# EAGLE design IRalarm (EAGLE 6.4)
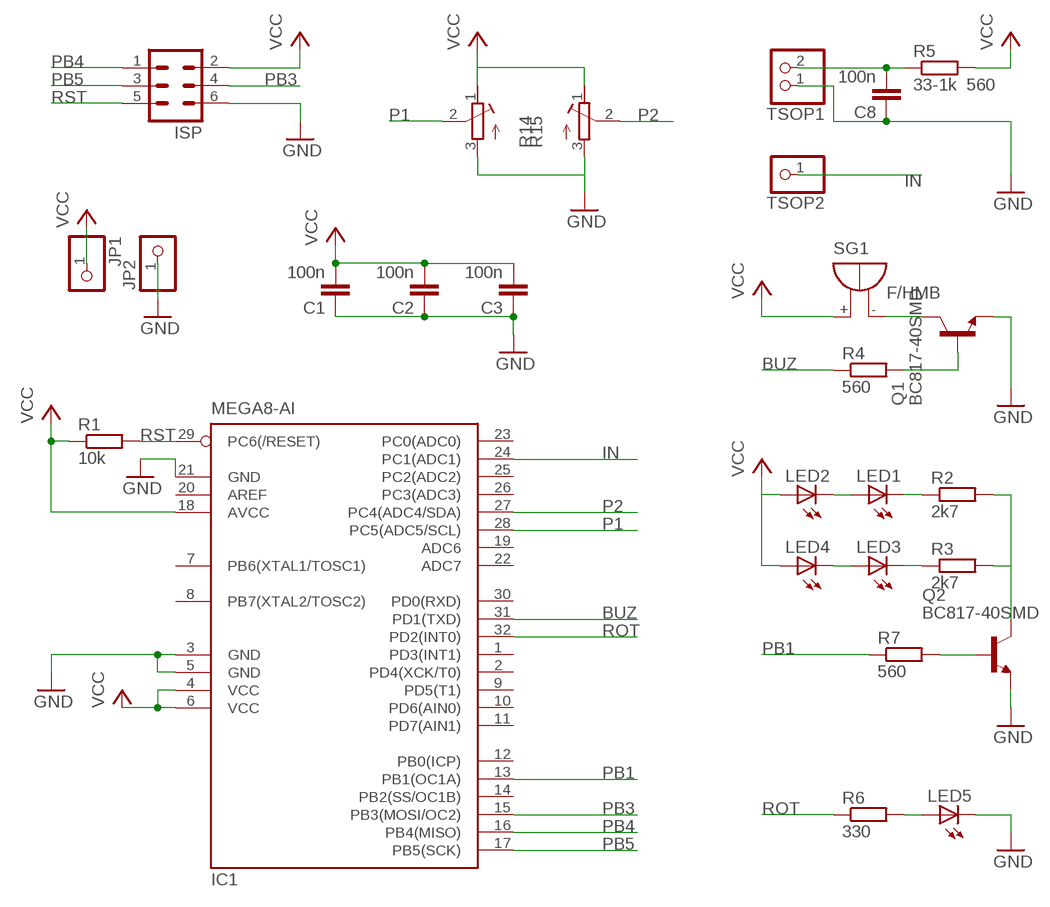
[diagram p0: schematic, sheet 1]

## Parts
C1  100n  C-EUC0805  [C0805]
C2  100n  C-EUC0805  [C0805]
C3  100n  C-EUC0805  [C0805]
C8  100n  C-EUC0805  [C0805]
IC1  MEGA8-AI  [TQFP32-08]
ISP  ML6  [ML6]
JP1  PINHD-1X1  [1X01]
JP2  PINHD-1X1  [1X01]
LED1  LED3MM  [LED3MM]
LED2  LED3MM  [LED3MM]
LED3  LED3MM  [LED3MM]
LED4  LED3MM  [LED3MM]
LED5  LED3MM  [LED3MM]
Q1  BC817-40SMD  [SOT23-BEC]
Q2  BC817-40SMD  [SOT23-BEC]
R1  10k  R-EU_R0805  [R0805]
R2  2k7  R-EU_R0805  [R0805]
R3  2k7  R-EU_R0805  [R0805]
R4  560  R-EU_R0805  [R0805]
R5  33-1k 560  R-EU_R0805  [R0805]
R6  330  R-EU_R0805  [R0805]
R7  560  R-EU_R0805  [R0805]
R14  R-TRIMM4G13  [RTRIM4G13]
R15  R-TRIMM4G13  [RTRIM4G13]
SG1  F/HMB  [F/HMB]
TSOP1  PINHD-1X2  [1X02]
TSOP2  PINHD-1X1  [1X01]

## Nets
BUZ: IC1.31(PD1(TXD)) R4.1
GND: C1.1 C2.1 C3.1 C8.1 IC1.3(GND) IC1.5(GND) IC1.21(GND) ISP.6 JP2.1 LED5.K(C) Q1.E Q2.E R14.3(A) R15.3(A) TSOP1.1
IN: IC1.24(PC1(ADC1)) TSOP2.1
N$1: LED1.K(C) R2.1
N$2: LED1.A LED2.K(C)
N$3: LED3.K(C) R3.1
N$4: LED5.A R6.2
N$5: LED3.A LED4.K(C)
N$6: Q2.C R2.2 R3.2
N$7: Q1.C SG1.-
N$8: Q2.B R7.2
N$9: C8.2 R5.1 TSOP1.2
N$10: Q1.B R4.2
P1: IC1.28(PC5(ADC5/SCL)) R14.2(S)
P2: IC1.27(PC4(ADC4/SDA)) R15.2(S)
PB1: IC1.13(PB1(OC1A)) R7.1
PB3: IC1.15(PB3(MOSI/OC2)) ISP.4
PB4: IC1.16(PB4(MISO)) ISP.1
PB5: IC1.17(PB5(SCK)) ISP.3
ROT: IC1.32(PD2(INT0)) R6.1
RST: IC1.29(PC6(/RESET)) ISP.5 R1.2
VCC: C1.2 C2.2 C3.2 IC1.4(VCC) IC1.6(VCC) IC1.18(AVCC) ISP.2 JP1.1 LED2.A LED4.A R1.1 R5.2 R14.1(E) R15.1(E) SG1.+
Unconnected: IC1.1(PD3(INT1)) IC1.2(PD4(XCK/T0)) IC1.7(PB6(XTAL1/TOSC1)) IC1.8(PB7(XTAL2/TOSC2)) IC1.9(PD5(T1)) IC1.10(PD6(AIN0)) IC1.11(PD7(AIN1)) IC1.12(PB0(ICP)) IC1.14(PB2(SS/OC1B)) IC1.19(ADC6) IC1.20(AREF) IC1.22(ADC7) IC1.23(PC0(ADC0)) IC1.25(PC2(ADC2)) IC1.26(PC3(ADC3)) IC1.30(PD0(RXD))

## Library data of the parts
C1-C3 C8 = rcl:C-EU: CAPACITOR, European symbol
IC1 = atmel:MEGA8: MICROCONTROLLER 8 Kbytes FLASH, 1 kbytes SRAM, 512 bytes EEPROM, USART, 6-channel 10 bit ADC, 2-channel 8 bit ADC Pin compatible with Atmega48, ATMega88, ATMega168 Source: avr.lbr
ISP = con-harting-ml:ML6: HARTING
JP1 JP2 TSOP2 = pinhead:PINHD-1X1: PIN HEADER
LED1-LED5 = led:LED: LED
Q1 Q2 = transistor-npn:BC817*: NPN Transistor
R1-R7 = rcl:R-EU_: RESISTOR, European symbol
R14 R15 = rcl:R-TRIMM: Trimm resistor
SG1 = buzzer:F/HMB: BUZZER; OC_FARNELL: unknown; OC_NEWARK: unknown
TSOP1 = pinhead:PINHD-1X2: PIN HEADER

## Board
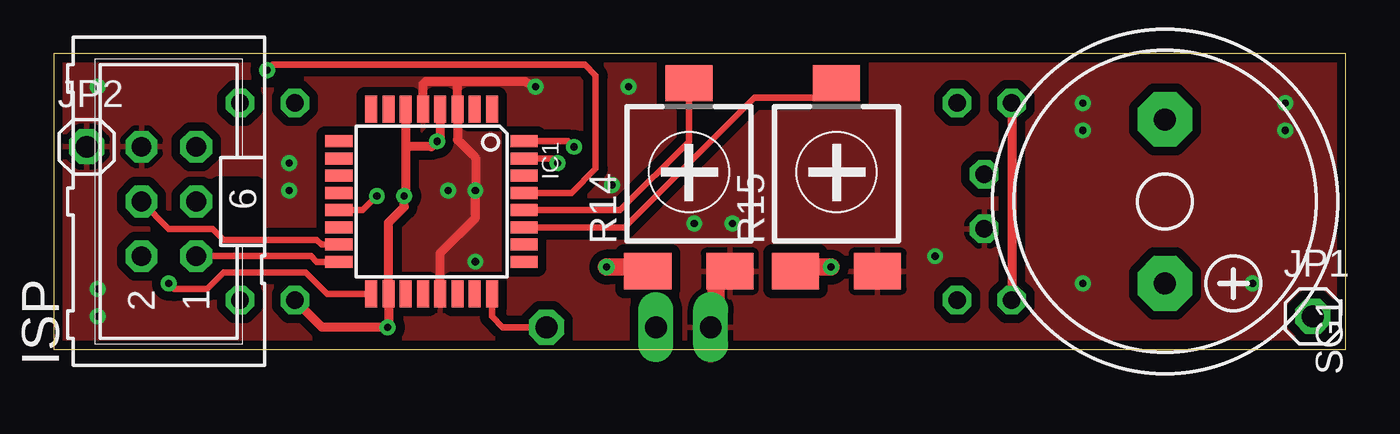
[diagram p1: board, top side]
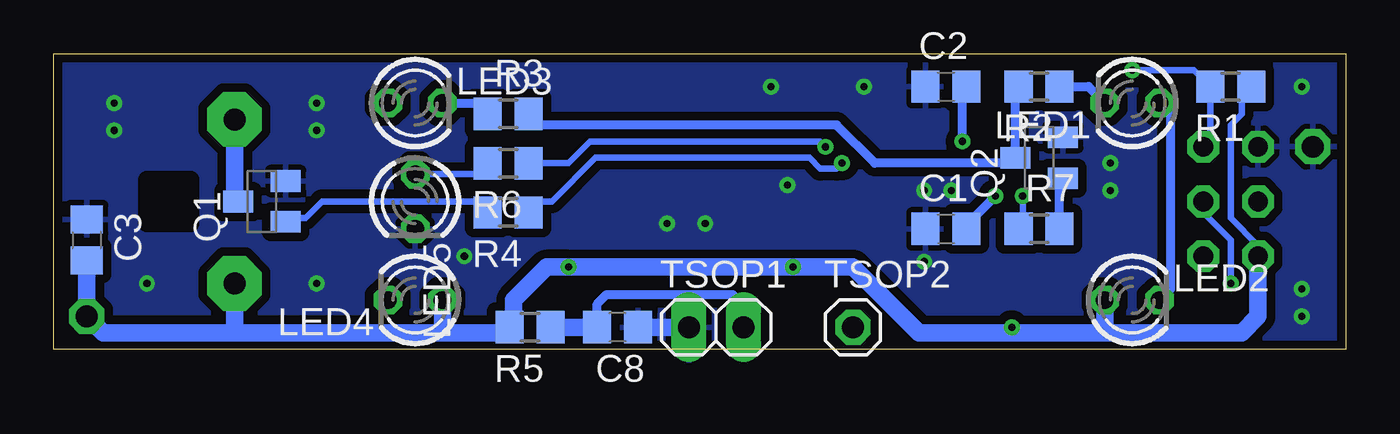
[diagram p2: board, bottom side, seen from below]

Size 59.94 x 13.72 mm. Coordinates in mm from the lower left corner, seen from the top.
Outline: 0,0 59.94,0 59.94,13.72 0,13.72 0,0
Copper layers (1*16): Top 0.035mm / dielectric 1.5mm / Bottom 0.035mm
Design rules "default *": minimum track width 10mil, minimum drill 24mil, track to track 8mil, track to pad 8mil, pad to pad 8mil, via to via 8mil, smd to smd 8mil, copper to edge 5mil, drill to drill 8mil, minimum pad ring 10mil, minimum via ring 8mil, stop-mask expansion 4mil, vias tented up to drill 15mil, thermal gap 10mil
tRestrict: area 7.6,5.8 to 9.4,7.6
bRestrict: area 53.6,5.8 to 55.6,7.9

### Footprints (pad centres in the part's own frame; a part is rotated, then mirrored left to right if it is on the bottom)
C0805 = smd 1.3 x 1.5: 1 -0.95,0; 2 0.95,0
TQFP32-08 = smd 1.27 x 0.559: 1 -4.293,2.8; 2 -4.293,2; 3 -4.293,1.2; 4 -4.293,0.4; 5 -4.293,-0.4; 6 -4.293,-1.2; 7 -4.293,-2; 8 -4.293,-2.8; 17 4.293,-2.8; 18 4.293,-2; 19 4.293,-1.2; 20 4.293,-0.4; 21 4.293,0.4; 22 4.293,1.2; 23 4.293,2; 24 4.293,2.8 | smd 0.559 x 1.27: 9 -2.8,-4.293; 10 -2,-4.293; 11 -1.2,-4.293; 12 -0.4,-4.293; 13 0.4,-4.293; 14 1.2,-4.293; 15 2,-4.293; 16 2.8,-4.293; 25 2.8,4.293; 26 2,4.293; 27 1.2,4.293; 28 0.4,4.293; 29 -0.4,4.293; 30 -1.2,4.293; 31 -2,4.293; 32 -2.8,4.293
ML6 = drill 0.914 octagon: 1 -2.54,-1.27; 2 -2.54,1.27; 3 0,-1.27; 4 0,1.27; 5 2.54,-1.27; 6 2.54,1.27
1X01 = drill 1.016 octagon: 1 0,0
LED3MM = drill 0.813 octagon: A -1.27,0; K 1.27,0
SOT23-BEC = smd 1 x 1.4: B -0.95,-1.1; C 0,1.1; E 0.95,-1.1
R0805 = smd 1.3 x 1.5: 1 -0.95,0; 2 0.95,0
RTRIM4G13 = smd 2.184 x 1.676: 1 -1.905,-4.763; 2 0,3.969; 3 1.905,-4.763
F/HMB = drill 1.016 pad 2.54 octagon: + 3.81,0; - -3.81,0
1X02 = drill 1.016 long: 1 -1.27,0; 2 1.27,0

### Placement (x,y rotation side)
C1  18.54,5.59 0 bottom
C2  18.54,12.19 0 bottom
C3  58.42,5.08 270 bottom
C8  33.78,1.02 180 bottom
IC1  17.53,6.86 270 top
ISP  5.33,6.86 90 top
JP1  58.42,1.52 0 top
JP2  1.52,9.4 0 top
LED1  9.91,11.43 180 bottom
LED2  9.91,2.29 0 bottom
LED3  43.18,11.43 0 bottom
LED4  43.18,2.29 180 bottom
LED5  43.18,6.86 270 bottom
Q1  50.29,6.86 90 bottom
Q2  14.22,8.89 90 bottom
R1  5.33,12.19 180 bottom
R2  14.22,12.19 180 bottom
R3  38.86,10.92 0 bottom
R4  38.86,6.35 180 bottom
R5  37.85,1.02 180 bottom
R6  38.86,8.64 180 bottom
R7  14.22,5.59 0 bottom
R14  29.46,8.38 0 top
R15  36.32,8.38 0 top
SG1  51.56,6.86 270 top
TSOP1  29.21,1.02 0 bottom
TSOP2  22.86,1.02 0 bottom

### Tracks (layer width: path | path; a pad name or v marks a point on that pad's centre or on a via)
BUZ  (via drill 0.33)
  Top 0.305: IC1.31 23.15,8.86 v23.37,8.64
  Bottom 0.305: v23.37,8.64 23.62,8.38 24.38,8.38 24.89,8.89 34.8,8.89 36.83,6.86 37.4,6.86 R4.1
GND  (via drill 0.33)
  Top 0.406: IC1.5 17.13,12.3 17.27,12.45 18.8,12.45 | 18.8,12.45 21.84,12.45 v22.35,12.19 | 18.8,12.45 18.73,12.38 IC1.3 18.73,9.72 19.56,8.89 v19.56,7.37 19.56,6.1 17.93,4.46 IC1.21
  Top 0.813: R14.3 31.3,3.62 30.73,3.05 30.73,1.27 TSOP1.1
  Bottom 0.813: C8.1 TSOP1.1
  other vias: 10.92,8.64 10.92,7.37 2.03,1.52 2.03,2.79 2.03,12.19 47.75,11.43 47.75,10.16 57.15,11.43 57.15,10.16 55.63,3.05 47.75,3.05 18.29,7.37 19.56,4.06 40.89,4.32 31.5,5.84 29.72,5.84 26.67,12.19 25.91,7.62
  pour Top (isolate 0.406): -0.51,14.22 60.45,14.22 60.45,-0.51 -0.51,-0.51
  pour Bottom (isolate 0.406): -0.51,14.22 60.45,14.22 60.45,-0.51 -0.51,-0.51
IN
  Top 0.305: IC1.24 20.33,1.52 20.83,1.02 TSOP2.1
N$1
  Bottom 0.406: R2.1 11.94,12.19 LED1.K
N$2
  Bottom 0.406: LED1.A 8.13,10.92 8.13,2.79 LED2.K
N$3
  Bottom 0.406: LED3.K 40.32,11.43 R3.1
N$4
  Bottom 0.305: LED5.A 40.32,8.13 R6.2
N$5
  Top 0.406: LED3.A LED4.K
N$6
  Bottom 0.406: R2.2 15.32,12.04 Q2.C 15.58,8.64 21.84,8.64 23.62,10.41 37.4,10.41 R3.2
N$7
  Bottom 0.813: SG1.- 51.56,7.03 Q1.C
N$8
  Bottom 0.406: R7.2 13.27,7.79 Q2.B
N$9
  Bottom 0.406: C8.2 34.73,2.1 34.29,2.54 28.45,2.54 27.94,2.03 TSOP1.2
  Bottom 0.813: R5.1 C8.2
N$10
  Bottom 0.305: Q1.B 49,6.1 48.26,6.1 47.5,6.86 40.32,6.86 R4.2
P1
  Top 0.305: IC1.28 26.27,6.46 29.46,9.65 R14.2
P2
  Top 0.305: IC1.27 26.49,5.66 32.51,11.68 35.66,11.68 R15.2
PB1  (via drill 0.33)
  Top 0.305: IC1.13 14.33,6.46 v14.99,7.11
  Bottom 0.305: v14.99,7.11 14.99,5.78 R7.1
PB3
  Top 0.305: IC1.15 12.41,4.86 12.19,5.08 7.87,5.08 7.37,5.59 5.33,5.59 ISP.4
PB4
  Top 0.305: IC1.16 12.2,4.06 11.94,4.32 ISP.1
PB5  (via drill 0.33)
  Top 0.305: IC1.17 12.68,2.56 11.68,3.56 7.87,3.56 7.11,2.79 5.59,2.79 v5.33,3.05
  Bottom 0.305: ISP.3 6.6,6.35 5.33,5.08 v5.33,3.05
ROT  (via drill 0.33)
  Top 0.305: IC1.32 23.87,9.66 v24.13,9.4
  Bottom 0.305: v24.13,9.4 24.38,9.65 35.05,9.65 36.07,8.64 R6.1
RST  (via drill 0.33)
  Top 0.305: v9.91,12.95 10.16,13.21 24.64,13.21 25.15,12.7 25.15,8.38 24.02,7.26 IC1.29
  Bottom 0.305: ISP.5 6.28,9.72 R1.2 7.05,12.95 v9.91,12.95
VCC  (via drill 0.33)
  Top 0.406: LED2.A 12.45,1.02 v15.49,1.02 15.53,1.05 IC1.18 15.53,5.87 16.26,6.6 v16.26,7.11 16.33,7.18 16.33,9.4 | IC1.4 17.93,9.8 v17.78,9.65 17.53,9.4 16.33,9.4 | IC1.6 16.33,9.4
  Top 0.813: R14.1 27.11,3.62 26.92,3.81 v25.65,3.81 | R15.1 34.86,3.62 35.05,3.81 v36.07,3.81
  Bottom 0.305: ISP.2 4.06,4.83 5.33,6.1 5.33,10.41 4.83,10.92 4.83,12 R1.1
  Bottom 0.406: v15.49,1.02 15.49,0.76 | 17.53,5.59 C1.2 17.59,5.78 v16.26,7.11 | v17.78,9.65 17.78,12 C2.2
  Bottom 0.813: 41.91,0.76 39.05,0.76 R5.2 38.61,1.2 38.61,2.29 37.08,3.81 v36.07,3.81 v25.65,3.81 22.86,3.81 19.81,0.76 15.49,0.76 11.43,0.76 | 41.91,0.76 51.56,0.76 | 51.56,0.76 57.66,0.76 JP1.1 C3.2 | SG1.+ 51.56,0.76 | ISP.2 4.06,1.52 4.83,0.76 11.43,0.76 | LED2.A 11.18,1.02 11.43,0.76 | LED4.A 41.91,0.76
